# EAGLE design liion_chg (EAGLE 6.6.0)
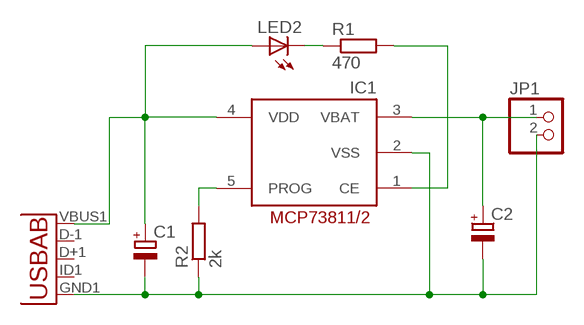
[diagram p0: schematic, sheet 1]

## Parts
C1  CPOL-EUB/3528-21W  [B/3528-21W]
C2  CPOL-EUB/3528-21W  [B/3528-21W]
IC1  MCP73811/2  [SOT23-5L]
JP1  PINHD-1X2  [1X02]
LED2  LEDCHIPLED_1206  [CHIPLED_1206]
R1  470  R-EU_M1206  [M1206]
R2  2k  R-EU_M1206  [M1206]
U1  USB-AB""  [USB-AB-MICRO-SMD_V02_BOSS]

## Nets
GND: C1.- C2.- IC1.2(VSS) JP1.2 R2.1 U1.GND1(GND)
N$1: IC1.5(PROG) R2.2
N$2: LED2.C R1.1
N$3: C1.+ IC1.4(VDD) LED2.A U1.VBUS1(VBUS)
N$4: C2.+ IC1.3(VBAT) JP1.1
N$5: IC1.1(CE) R1.2
Unconnected: U1.D+1(D+) U1.D-1(D-) U1.ID1(USBID)

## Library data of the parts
C1 C2 = rcl:CPOL-EU: POLARIZED CAPACITOR, European symbol
IC1 = adafruit:MCP73811/2: MCP73811 and MCP73812 Simple, Miniature Single-Cell, Fully Integrated Li-Ion / Li-Polymer Charge Management Controllers SOT-23-5 package, no indicator LED but with adjustable current, small and very inexpensive
JP1 = pinhead:PINHD-1X2: PIN HEADER
LED2 = led:LED: LED
R1 R2 = resistor:R-EU_: RESISTOR, European symbol
U1 = Testing:USB-AB: This is a USB AB connector that is compatible with USB OTG. i.e. this connector can serve as a host or device

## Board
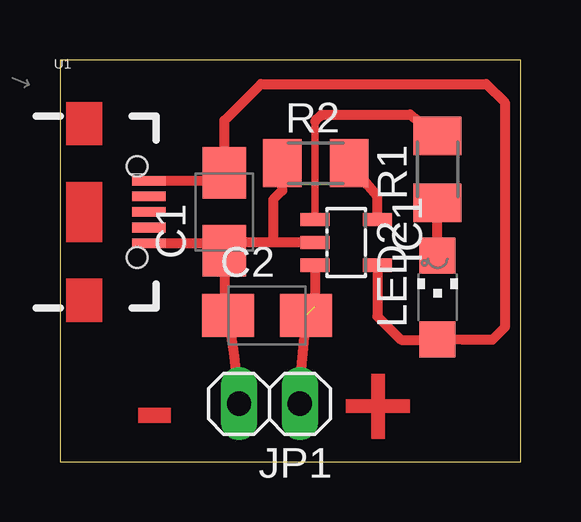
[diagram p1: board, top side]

Size 19.23 x 16.75 mm. Coordinates in mm from the lower left corner, seen from the top.
Outline: 0,0 19.23,0 19.23,16.75 0,16.75 0,0
Copper layers (1*16): Top 0.035mm / dielectric 1.5mm / Bottom 0.035mm
Design rules "default": minimum track width 10mil, minimum drill 24mil, track to track 8mil, track to pad 8mil, pad to pad 8mil, via to via 8mil, smd to smd 8mil, copper to edge 40mil, drill to drill 8mil, minimum pad ring 10mil, minimum via ring 8mil, stop-mask expansion 4mil, vias tented up to drill 0mil, thermal gap 10mil

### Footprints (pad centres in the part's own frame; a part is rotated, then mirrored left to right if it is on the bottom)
B/3528-21W = smd 2.15 x 1.8: + 1.625,0; - -1.625,0
SOT23-5L = smd 0.55 x 1.2: 1 -0.95,-1.3; 2 0,-1.3; 3 0.95,-1.3; 4 0.95,1.3; 5 -0.95,1.3
1X02 = drill 1.016 long: 1 -1.27,0; 2 1.27,0
CHIPLED_1206 = smd 1.5 x 1.5: A 0,-1.75; C 0,1.75
M1206 = smd 1.6 x 2: 1 -1.4,0; 2 1.4,0
USB-AB-MICRO-SMD_V02_BOSS = smd 1.4 x 0.4: D+1 2.7,0; D-1 2.7,0.65; GND1 2.7,-1.3; ID1 2.7,-0.65; VBUS1 2.7,1.3 | hole 0.85: 2.2,1.9; 2.2,-1.9

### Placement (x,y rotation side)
C1  6.86,10.41 90 top
C2  8.64,6.1 0 top
IC1  11.94,9.14 270 top
JP1  8.74,2.41 180 top
LED2  15.75,6.86 0 top
R1  15.75,12.19 90 top
R2  10.67,12.45 0 top
U1  1.02,10.41 0 top

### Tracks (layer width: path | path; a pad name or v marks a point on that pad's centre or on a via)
GND
  Top 0.406: U1.GND1 6.53,9.11 C1.- | IC1.2 8.89,9.14 | 8.89,9.14 7.21,9.14 C1.- | C1.- 6.86,6.25 C2.- 7.26,4.39 JP1.2 | R2.1 9.27,11.3 8.89,10.92 8.89,9.14
N$1
  Top 0.406: IC1.5 13.24,11.08 R2.2
N$2
  Top 0.406: LED2.C R1.1
N$3
  Top 0.406: U1.VBUS1 6.53,11.71 C1.+ 6.86,14.22 8.38,15.75 17.78,15.75 18.54,14.99 18.54,5.59 18.03,5.08 16.79,5.08 LED2.A 15.72,5.08 14.22,5.08 13.24,6.07 IC1.4
N$4  (1 unrouted)
  Top 0.406: IC1.3 10.64,6.47 | C2.+ 10.01,3.43 JP1.1
N$5
  Top 0.305: IC1.1 10.64,14.19
  Top 0.406: 10.64,14.19 10.92,14.48 14.61,14.48 R1.2

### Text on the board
Top: - | +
